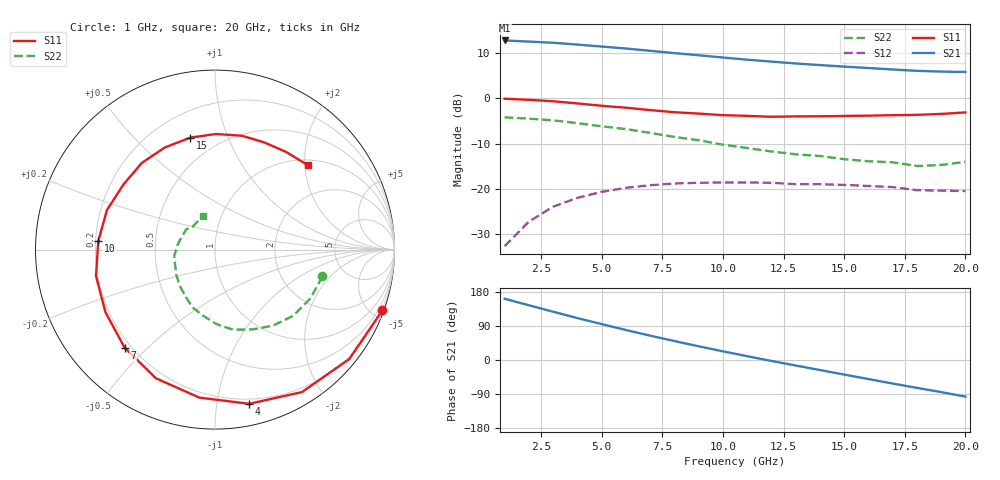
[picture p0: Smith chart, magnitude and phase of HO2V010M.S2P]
! SIEMENS Small Signal Semiconductors
! CFY67-10
! GaAs HEMT in Micro-X
! VDS = 2 V  ID = 10 mA
! Common Source S-Parameters:  August  1993
# GHz  S  MA  R  50
!  f  S11  S21  S12  S22
! GHz  MAG  ANG  MAG  ANG  MAG  ANG  MAG  ANG
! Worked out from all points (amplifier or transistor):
!   20 points, 1 GHz to 20 GHz, reference 50 ohm
!   highest |S21| = 12.9 dB at 1 GHz (marker M1)
!   |S21| within 3 dB of that: start of sweep to 8.404 GHz
!   unconditionally stable (mu >= 1): 12.4 GHz to end of sweep
!   at 4 GHz: K = 0.34, MSG = 17.0 dB, |S12| = -22.0 dB
!   at 11 GHz: K = 0.89, MSG = 13.6 dB, |S12| = -18.6 dB
!   at 20 GHz: K = 1.29, MAG = 10.0 dB, |S12| = -20.5 dB
!   lowest NFmin = 0.39 dB at 2 GHz
!   S11 on the Smith chart (normalised r, x): 1 GHz: 0.13, -5.67; 4 GHz: 0.16, -1.23; 7 GHz: 0.17, -0.43; 10 GHz: 0.21, +0.03; 15 GHz: 0.35, +0.74; 20 GHz: 1.13, +2.08
1  0.992 -20.0  4.394 161.6  0.023 76.6  0.617 -14.0
2  0.965 -39.2  4.269 144.5  0.043 63.6  0.597 -27.1
3  0.93 -58.6  4.141 127.4  0.063 50.6  0.571 -40.3
4  0.88 -77.5  3.955 110.6  0.079 38.6  0.532 -52.9
5  0.829 -96.1  3.762 94.8  0.092 27.3  0.491 -64.9
6  0.789 -114.6  3.576 79.2  0.102 16.4  0.457 -77.4
7  0.743 -132.7  3.372 64.3  0.109 5.9  0.415 -88.9
8  0.703 -150.3  3.181 50.0  0.114 -3.4  0.374 -100.3
9  0.679 -167.5  3.01 36.2  0.116 -12.3  0.344 -111.8
10  0.652 175.9  2.843 22.9  0.117 -21.0  0.307 -122.5
11  0.641 159.9  2.69 10.1  0.117 -28.8  0.282 -134.1
12  0.626 144.5  2.562 -2.5  0.116 -36.5  0.258 -146.4
13  0.632 130.1  2.441 -14.5  0.112 -41.4  0.24 -157.3
14  0.634 116.2  2.344 -26.4  0.112 -50.1  0.23 -170.9
15  0.639 102.4  2.253 -38.5  0.11 -57.6  0.212 174.2
16  0.644 89.5  2.174 -50.2  0.107 -65.1  0.201 162.7
17  0.652 76.7  2.094 -62.2  0.104 -72.0  0.196 144.8
18  0.657 65.4  2.023 -73.5  0.096 -78.7  0.178 134.6
19  0.673 54.0  1.984 -84.7  0.095 -83.9  0.183 123.6
20  0.7 42.1  1.965 -96.6  0.094 -90.9  0.198 109.1
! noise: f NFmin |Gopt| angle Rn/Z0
2  0.39  0.77  27  0.31
4  0.51  0.73  55  0.25
6  0.59  0.69  84  0.17
8  0.69  0.64  116  0.09
10  0.78  0.6  148  0.04
12  0.87  0.57  -179  0.02
14  0.97  0.55  -147  0.05
16  1.06  0.54  -116  0.12
18  1.15  0.54  -87  0.23
20  1.24  0.53  -60  0.35
